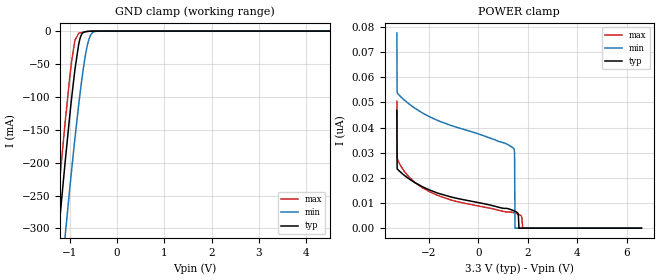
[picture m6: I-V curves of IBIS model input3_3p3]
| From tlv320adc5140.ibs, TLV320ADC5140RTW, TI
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|   input3_3p3 Model
[Model]   input3_3p3
Model_type   Input
Vinl = 0.8
Vinh = 2
|   typ   min   max
C_comp   1.5123pF   1.4245pF   1.5909pF
| Where Nom  PVT is Nominal Process, 3.3V, 27C
|   Fast PVT is Strong Process,  3.6V, -40C
|   Slow PVT is Weak Process,   3.0V, 150C
[Voltage Range]   3.3   3   3.6
|Junction Temperature
[Temperature Range]   27   150   -40
[Power Clamp Reference]   3.3   3   3.6
[GND Clamp Reference]   0   0   0
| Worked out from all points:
|   GND clamp passes 1 mA (typ) near -0.68 V on its own axis
[GND Clamp]
|   Voltage   I(typ)   I(min)   I(max)
-3.3V     -2.018A    -2.044A    -2.005A
-1.31V    -362.8mA   -474.1mA   -303.2mA
-1.261V   -323.2mA   -434.9mA   -263.2mA
-1.211V   -284.1mA   -396.2mA   -223.8mA
-1.092V   -193.1mA   -305.3mA   -132.8mA
-963.6mV  -102mA     -211.5mA   -46.24mA
-894.3mV  -59mA      -163.8mA   -14.13mA
-815.1mV  -20.65mA   -112.9mA   -3.346mA
-745.8mV  -4.384mA   -72.75mA   -2.125mA
-636.9mV  -528.4uA   -23.82mA   -720.5uA
-468.6mV  -8.975uA   -661.8uA   -8.367uA
6.6V      0A         0A         0A
[POWER Clamp]
|   Voltage   I(typ)   I(min)   I(max)
-3.3V     46.82nA    77.59nA    50.44nA
-3.29V    23.65nA    53.97nA    27.83nA
-2.785V   19.44nA    49.2nA     20.05nA
-1.092V   12.35nA    40.75nA    11.14nA
1.442V    6.892nA    31.49nA    6.101nA
1.462V    6.808nA    29.93nA    6.044nA
1.482V    6.72nA     0A         5.984nA
1.601V    5.914nA    0A         5.582nA
1.64V     0A         0A         5.425nA
1.749V    0A         0A         4.634nA
1.789V    0A         0A         0A
6.6V      0A         0A         0A
